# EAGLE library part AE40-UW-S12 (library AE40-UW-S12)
Isolated DC/DC Converters - Through Hole 200-1500Vin12V 3.33A 40W Iso Reg DIP Source: Datasheet
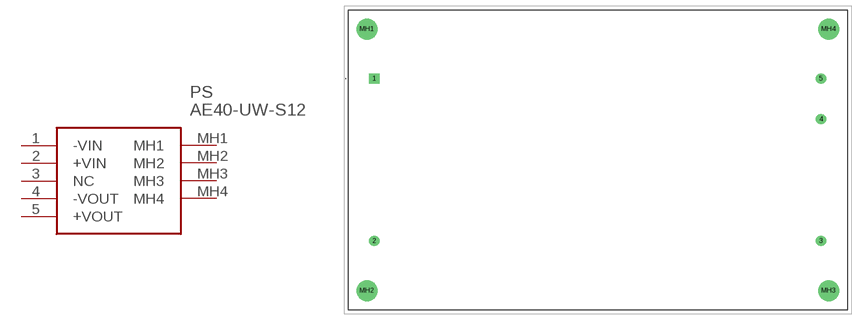
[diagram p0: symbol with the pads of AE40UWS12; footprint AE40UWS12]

Designator prefix PS

## AE40-UW-S12 (Arrow_Part_Number: AE40-UW-S12; Arrow_Price-Stock: https://www.arrow.com/en/products/ae40-uw-s12/cui-inc; Description: Isolated DC/DC Converters - Through Hole 200-1500Vin12V 3.33A 40W Iso Reg DIP; Height: 40.5mm; Manufacturer_Name: CUI Inc.; Manufacturer_Part_Number: AE40-UW-S12; Mouser_Part_Number: 490-AE40-UW-S12; Mouser_Price-Stock: https://www.mouser.co.uk/ProductDetail/CUI-Inc/AE40-UW-S12?qs=f9yNj16SXrIfTv9jjRHLaw%3D%3D)  [AE40UWS12]
1  -VIN
2  +VIN
3  NC  nc
4  -VOUT
5  +VOUT
MH1  MH1
MH2  MH2
MH3  MH3
MH4  MH4

## Footprint AE40UWS12 (pad centres in mm)
AE40-UW-S12-1
drill 1.7 pad 2.55 square: 1 0,0
drill 1.7 pad 2.55: 2 0,-40.64; 3 111.76,-40.64; 4 111.76,-10.16; 5 111.76,0
drill 3.5 pad 5.25: MH1 -1.87,12.43; MH2 -1.87,-53.07; MH3 113.63,-53.07; MH4 113.63,12.43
